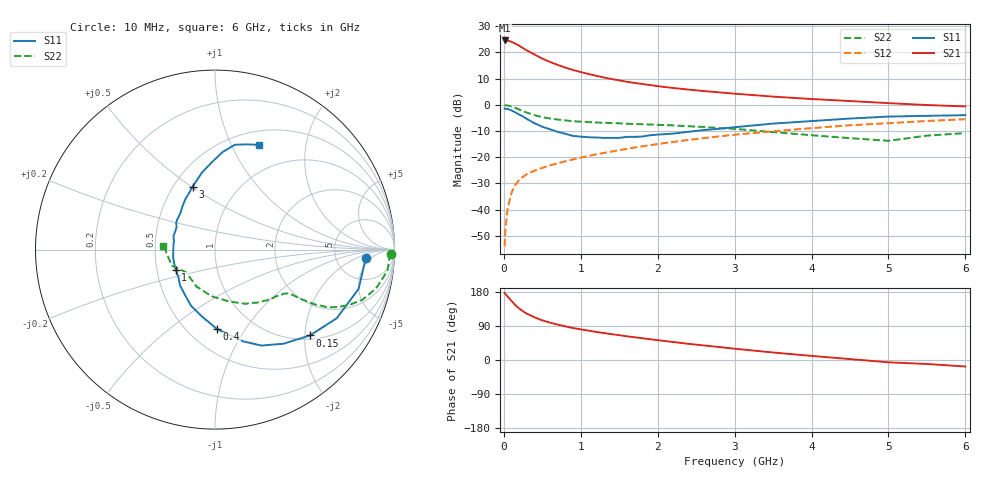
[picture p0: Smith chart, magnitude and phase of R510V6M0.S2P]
! SIEMENS Small Signal Semiconductors
! BFR183
! Si NPN RF Bipolar Junction Transistor in SOT23
! VCE = 10 V  IC = 6 mA
! Common Emitter S-Parameters:  May  1996
# GHz  S  MA  R  50
!  f  S11  S21  S12  S22
! GHz  MAG  ANG  MAG  ANG  MAG  ANG  MAG  ANG
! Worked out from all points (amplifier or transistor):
!   36 points, 10 MHz to 6 GHz, reference 50 ohm
!   highest |S21| = 24.5 dB at 10 MHz (marker M1)
!   |S21| within 3 dB of that: start of sweep to 253.1 MHz
!   unconditionally stable (mu >= 1): 1.015 GHz to 2.758 GHz
!   at 250 MHz: K = 0.45, MSG = 24.5 dB, |S12| = -27.5 dB
!   at 1.4 GHz: K = 1.05, MAG = 12.4 dB, |S12| = -17.9 dB
!   at 6 GHz: K = 0.88, MSG = 2.4 dB, |S12| = -5.5 dB
!   S11 on the Smith chart (normalised r, x): 10 MHz: 11, -3; 150 MHz: 1.09, -2.12; 400 MHz: 0.69, -0.76; 1 GHz: 0.63, -0.15; 3 GHz: 0.62, +0.50; 6 GHz: 0.66, +1.28
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0.01  0.8434 -3.1  16.84 177.2  0.002 79.9  0.9813 -1.4
0.02  0.8355 -5.9  16.67 174.4  0.0041 91.6  0.9738 -2.8
0.05  0.8295 -15.3  16.75 167.2  0.0107 80.8  0.9677 -7.1
0.1  0.7787 -29.4  15.86 155.8  0.021 75.9  0.9224 -13.6
0.15  0.7134 -42.1  14.6 144.6  0.0298 69.0  0.8683 -18.7
0.2  0.6489 -53.9  13.37 135.8  0.0368 64.9  0.8085 -22.5
0.25  0.5938 -64.2  11.99 128.4  0.0423 62.1  0.7517 -25.2
0.3  0.5344 -73.0  10.85 122.2  0.0474 60.4  0.7086 -27.0
0.4  0.443 -88.5  9.053 112.5  0.0552 58.8  0.6326 -28.8
0.5  0.38 -101.0  7.581 104.5  0.0624 58.2  0.5789 -29.5
0.6  0.3404 -113.1  6.55 98.6  0.0697 58.0  0.5462 -29.9
0.8  0.2793 -134.1  5.104 88.7  0.0837 58.7  0.5027 -30.3
1  0.2462 -152.7  4.201 80.8  0.0976 59.8  0.4747 -30.9
1.1  0.2398 -162.5  3.862 77.6  0.1051 60.4  0.4657 -31.7
1.3  0.2324 -177.6  3.307 71.2  0.1203 59.9  0.452 -33.1
1.6  0.2436 161.7  2.741 62.5  0.1441 59.5  0.4345 -36.4
2.2  0.281 133.1  2.088 47.5  0.1948 56.9  0.4033 -44.6
3  0.372 109.6  1.625 29.8  0.2674 50.2  0.3467 -60.6
3.5  0.4365 99.5  1.428 19.8  0.3111 44.8  0.3003 -74.5
4.5  0.5447 85.6  1.176 2.4  0.406 33.5  0.2301 -116.6
5.5  0.6135 72.9  0.986 -10.5  0.4895 21.9  0.257 -159.7
6  0.6321 67.3  0.929 -17.2  0.5289 14.1  0.2878 175.7
